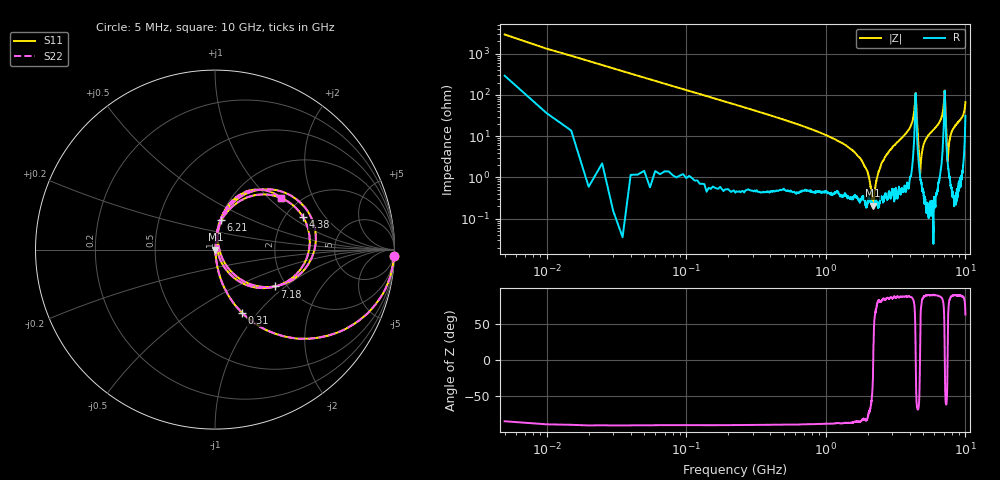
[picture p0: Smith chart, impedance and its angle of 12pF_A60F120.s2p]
! Amotech Co.,Ltd.
! http://www.amotech.co.kr/
! Part Number: A60F120
! These Parameters are Measured in Series Mode Connection
! Operation Temp=25[degC], DC Bias Voltage=0[V]
! Freq. Start=5[MHz] Stop=10[GHz], 2000[Steps]
! Date: Monday, July 20, 2020, 03:34:42
# GHZ S RI R 50.000000
!Freq.(Hz) S11(Real) S11(Imag) S21(Real) S21(Imag) S12(Real) S12(Imag) S22(Real) S22(Imag)
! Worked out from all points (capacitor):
!   2000 points, 5 MHz to 10 GHz, reference 50 ohm
!   read as one part in series: C = 12.1 pF near 55 MHz
!   lowest |Z| = 206 mohm at 2.175 GHz (marker M1)
!   series resonance near 2.187 GHz, so ESL is about 440 pH
!   S11 on the Smith chart (normalised r, x): 5 MHz: 7, -58; 310 MHz: 1.01, -0.84; 4.38 GHz: 2.47, +1.25; 6.21 GHz: 1.01, +0.35; 7.18 GHz: 1.73, -0.84; 10 GHz: 1.62, +1.19
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0.005  0.9954 -0.0338  0.00457 0.0338  0.00457 0.0338  0.9954 -0.0338
0.1  0.6322 -0.4785  0.3678 0.4785  0.3678 0.4785  0.6322 -0.4785
0.31  0.1516 -0.3529  0.8484 0.3529  0.8484 0.3529  0.1516 -0.3529
1.675  0.00458 -0.0345  0.9954 0.0345  0.9954 0.0345  0.00458 -0.0345
1.985  0.00255 -0.0138  0.9974 0.0138  0.9974 0.0138  0.00255 -0.0138
2.175  0.00185 -0.000893  0.9982 0.000893  0.9982 0.000893  0.00185 -0.000893
2.525  0.00384 0.0228  0.9962 -0.0228  0.9962 -0.0228  0.00384 0.0228
3.34  0.0118 0.0761  0.9882 -0.0761  0.9882 -0.0761  0.0118 0.0761
4.165  0.0645 0.2059  0.9355 -0.2059  0.9355 -0.2059  0.0645 0.2059
4.38  0.4899 0.183  0.5101 -0.183  0.5101 -0.183  0.4899 0.183
4.47  0.2209 -0.2103  0.7791 0.2103  0.7791 0.2103  0.2209 -0.2103
4.725  0.0116 -0.000423  0.9884 0.000423  0.9884 0.000423  0.0116 -0.000423
5.005  0.00814 0.0605  0.9919 -0.0605  0.9919 -0.0605  0.00814 0.0605
6.21  0.0332 0.1675  0.9668 -0.1675  0.9668 -0.1675  0.0332 0.1675
6.67  0.0748 0.2336  0.9252 -0.2336  0.9252 -0.2336  0.0748 0.2336
7.01  0.3443 0.3307  0.6557 -0.3307  0.6557 -0.3307  0.3443 0.3307
7.1  0.5615 0.0787  0.4385 -0.0787  0.4385 -0.0787  0.5615 0.0787
7.18  0.3318 -0.2054  0.6682 0.2054  0.6682 0.2054  0.3318 -0.2054
7.465  0.0227 0.00608  0.9773 -0.00608  0.9773 -0.00608  0.0227 0.00608
7.775  0.0171 0.0931  0.9829 -0.0931  0.9829 -0.0931  0.0171 0.0931
8.335  0.0305 0.1641  0.9695 -0.1641  0.9695 -0.1641  0.0305 0.1641
10  0.3672 0.2866  0.6328 -0.2866  0.6328 -0.2866  0.3672 0.2866
